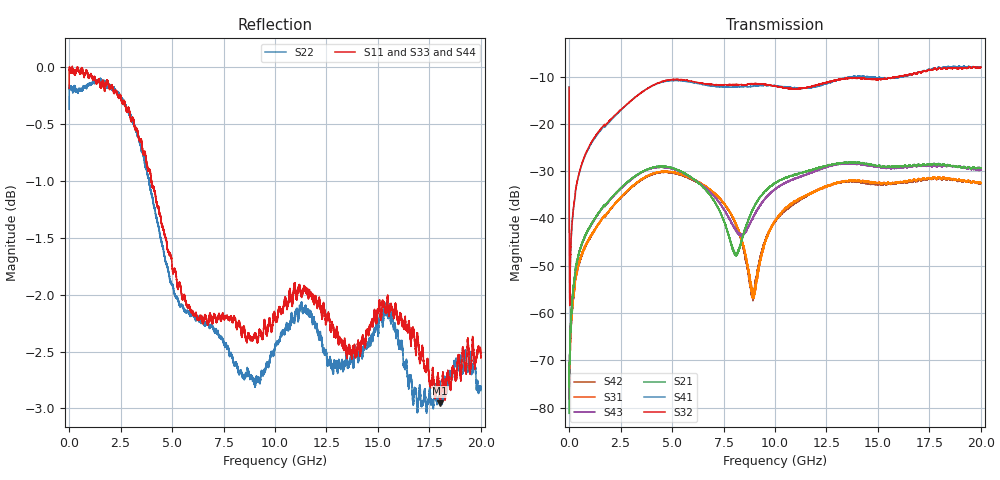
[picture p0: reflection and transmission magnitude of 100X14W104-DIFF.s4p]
!{100X14W104}
!Johanson Technology Inc.
!www.johansontechnology.com
!Test Board Conditions:
!Substrate Type  RO4350B
!Substrate Thickness  10 mil
!Substrate Dk  3.66
!TL Type: GCPW
!TL Trace Width  20 mil
!TL Gap  15 mil
!PART MODE DIFFERENTIAL
!DUT TOPOLOGY	DIFFERENTIAL 4-PORT
!Mounting Pad LxW  20x35 mil
# MHz S  dB  R 50
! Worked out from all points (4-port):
!   20001 points, 300 kHz to 20 GHz, reference 50 ohm
!   strongest paths, dB at 300 kHz, 5 GHz, 10 GHz, 15 GHz, 20 GHz:
!     S32: -12.3, -10.7, -12.0, -10.7, -8.0
!     S41: -12.2, -10.9, -11.9, -10.3, -8.0
!     S21: -81.2, -29.3, -32.5, -28.9, -29.3
!     S43: -74.0, -29.5, -33.8, -29.1, -29.8
!     S31: -71.4, -30.2, -40.5, -32.5, -32.5
!     S42: -74.6, -30.4, -40.6, -32.8, -32.6
!   lowest |S11| = -3.0 dB at 18.02 GHz (marker M1), VSWR 5.94, Z = 20.3 + j57.4 ohm
!   |S11| at or under -10 dB: nowhere
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0.3  -0.18 -165.7  -71.56 33.5  -77.98 20.9  -12.19 -75.2
     -81.18 -30.1  -0.37 -166.7  -12.31 -75.1  -70.79 -9.2
     -71.36 -19.5  -12.29 -75.7  -0.23 -165.5  -74.42 -44.9
     -12.16 -75.1  -74.63 10.1  -74.05 -9.5  -0.25 -165.9
106.298  -0.04 178.8  -60.00 71.0  -62.33 71.7  -43.71 71.8
         -60.04 70.3  -0.19 178.8  -43.51 71.6  -61.56 64.1
         -61.32 68.6  -43.74 72.2  -0.03 178.9  -59.98 68.2
         -43.76 71.4  -62.25 73.5  -60.16 76.6  -0.02 178.8
599.291  -0.01 173.6  -45.40 74.6  -47.73 71.3  -28.86 75.9
         -45.66 75.0  -0.20 172.4  -28.75 75.4  -48.00 70.4
         -47.82 71.5  -28.71 75.3  -0.09 172.4  -45.70 72.7
         -28.85 75.6  -48.12 69.4  -45.53 73.4  -0.10 172.2
3487.248  -0.64 155.3  -30.25 40.9  -31.78 33.4  -13.43 53.5
          -30.25 40.6  -0.69 155.6  -13.47 53.0  -31.95 33.8
          -31.85 33.8  -13.46 53.2  -0.58 155.4  -30.37 42.5
          -13.43 53.5  -31.96 33.8  -30.34 42.2  -0.65 157.1
8950.166  -2.38 128.3  -37.83 60.2  -56.18 -28.9  -12.06 -3.6
          -37.82 60.2  -2.74 130.7  -11.52 -6.2  -55.99 -17.2
          -55.55 -31.2  -11.52 -6.4  -2.43 130.5  -39.76 49.4
          -12.06 -3.7  -56.73 -11.9  -39.72 47.8  -2.36 135.4
18015.03  -2.95 78.1  -28.50 -33.8  -31.42 -70.7  -8.04 -28.4
          -28.61 -33.9  -2.78 81.9  -8.27 -32.0  -31.55 -67.0
          -31.43 -69.6  -8.22 -31.5  -2.50 81.3  -28.67 -27.2
          -8.14 -28.0  -31.39 -66.5  -28.80 -27.8  -2.62 89.9
20000  -2.54 66.7  -29.36 -43.7  -32.48 -83.1  -8.00 -38.5
       -29.32 -43.7  -2.84 69.5  -8.07 -40.4  -32.53 -80.1
       -32.47 -82.3  -8.05 -39.4  -2.71 67.0  -29.69 -41.5
       -8.02 -38.0  -32.59 -80.2  -29.82 -42.3  -2.54 71.1
